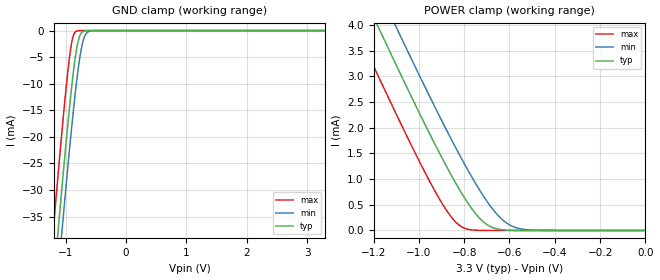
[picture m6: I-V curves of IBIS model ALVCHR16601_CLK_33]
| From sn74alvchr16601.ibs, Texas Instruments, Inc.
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[Model]   ALVCHR16601_CLK_33
Model_type  Input
Vinl=0.8
Vinh=2.0
| variable   typ   min   max
C_comp   2.03pF   1.65pF   2.56pF
[Temperature Range]   40   100   -40
| Ambient temperature   25   85   -40
[Voltage range]   3.3   3   3.6
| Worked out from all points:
|   GND clamp passes 1 mA (typ) near -0.77 V on its own axis
|   POWER clamp passes 1 mA (typ) near -0.85 V on its own axis
[GND Clamp]
| ALVCHR16601_CLK_33
|   Voltage   I(typ)   I(min)   I(max)
-3.3V     -341.8mA   -349.3mA   -332.6mA
-1.215V   -49.64mA   -57.94mA   -39mA
-1.185V   -45.67mA   -53.97mA   -35.01mA
-1.125V   -37.81mA   -46.1mA    -27.15mA
-1.065V   -30.11mA   -38.36mA   -19.53mA
-920mV    -12.76mA   -20.55mA   -3.721mA
-875mV    -8.132mA   -15.46mA   -1.066mA
-825mV    -3.926mA   -10.27mA   -137.3uA
-775mV    -1.292mA   -5.835mA   -13.58uA
-715mV    -205.6uA   -2.13mA    -809.3nA
-585mV    -2.268uA   -70.89uA   -1.785nA
3.3V      6.304pA    9.26pA     5.93pA
[POWER Clamp]
| ALVCHR16601_CLK_33
|   Voltage   I(typ)   I(min)   I(max)
-3.3V     24.83mA    25.52mA    23.96mA
-1.275V   4.872mA    5.61mA     3.918mA
-1.185V   4.018mA    4.758mA    3.062mA
-1.105V   3.269mA    4.008mA    2.314mA
-1.07V    2.945mA    3.683mA    1.992mA
-940mV    1.776mA    2.501mA    856.4uA
-845mV    982.9uA    1.676mA    200.1uA
-795mV    611.2uA    1.266mA    38.41uA
-725mV    207uA      738.7uA    1.527uA
-625mV    11.21uA    186.8uA    11.91nA
-510mV    181.6nA    9.688uA    52.91pA
-48.03fV  6.303pA    7.801pA    6.677pA
